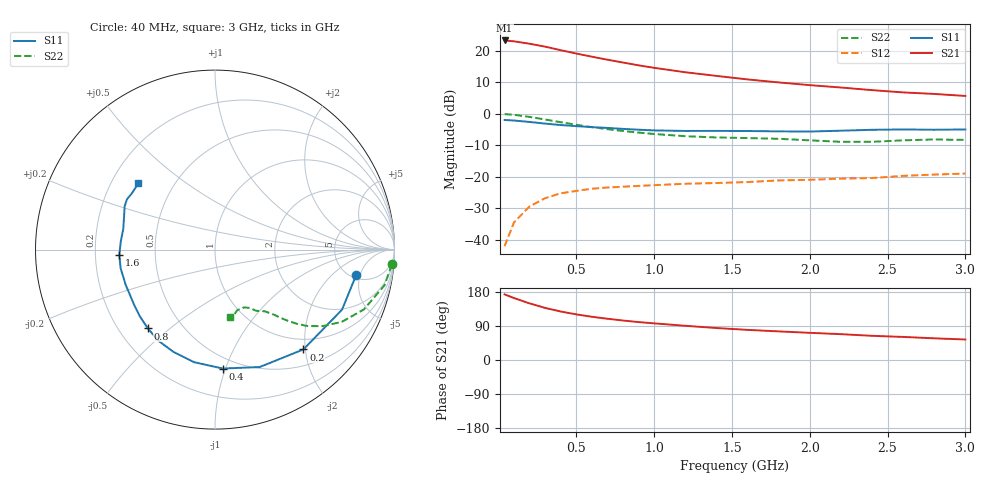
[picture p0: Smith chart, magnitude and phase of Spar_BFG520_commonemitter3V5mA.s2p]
! Filename:  BFG520B.S2P  Version:  2.1
! NXP part #: BFG520  Date: Feb 1992
! Bias condition: Vce=3V, Ic=5mA
! IN LINE PINNING: same data as with cross emitter pinning.
#  MHz  S  MA  R  50
! Freq  S11  S21  S12  S22  !GUM [dB]
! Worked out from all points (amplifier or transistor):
!   21 points, 40 MHz to 3 GHz, reference 50 ohm
!   highest |S21| = 23.2 dB at 40 MHz (marker M1)
!   |S21| within 3 dB of that: start of sweep to 393.2 MHz
!   unconditionally stable (mu >= 1): 1.746 GHz to end of sweep
!   at 300 MHz: K = 0.19, MSG = 24.0 dB, |S12| = -26.7 dB
!   at 1 GHz: K = 0.65, MSG = 18.6 dB, |S12| = -22.6 dB
!   at 3 GHz: K = 1.30, MAG = 9.0 dB, |S12| = -18.9 dB
!   lowest NFmin = 0.90 dB at 500 MHz
!   S11 on the Smith chart (normalised r, x): 40 MHz: 5.47, -4.32; 200 MHz: 0.79, -1.96; 400 MHz: 0.41, -0.98; 800 MHz: 0.32, -0.42; 1.6 GHz: 0.30, -0.03; 3 GHz: 0.31, +0.34
40  0.799 -10.3  14.52 173.1  0.008 84.1  0.989 -4.8
100  0.783 -25.3  14.07 163.5  0.019 77.0  0.965 -11.9
200  0.743 -48.5  12.89 149.4  0.034 66.6  0.894 -21.9
300  0.7 -69.2  11.59 137.5  0.046 58.1  0.813 -29.7
400  0.664 -86.3  10.19 128.0  0.055 52.3  0.736 -35.4
500  0.638 -100.5  9.02 120.4  0.06 47.6  0.67 -39.5
600  0.615 -112.1  8.033 114.1  0.065 44.7  0.615 -42.2
700  0.598 -121.7  7.204 108.9  0.068 42.6  0.571 -44.2
800  0.577 -130.4  6.491 104.2  0.07 41.7  0.535 -45.8
900  0.56 -138.4  5.868 100.1  0.072 41.1  0.504 -47.1
1000  0.546 -145.4  5.356 96.7  0.074 40.9  0.479 -48.4
1200  0.535 -158.4  4.556 90.3  0.078 40.6  0.442 -51.1
1400  0.536 -168.8  3.989 84.4  0.08 41.1  0.422 -54.0
1600  0.534 -176.7  3.507 79.5  0.083 43.4  0.413 -55.8
1800  0.527 175.3  3.144 75.5  0.088 44.4  0.402 -56.9
2000  0.524 167.1  2.847 71.7  0.09 46.6  0.38 -58.8
2200  0.54 159.7  2.61 68.2  0.094 47.7  0.36 -63.5
2400  0.558 154.5  2.372 63.8  0.096 50.1  0.36 -69.8
2600  0.565 150.3  2.183 60.9  0.104 51.9  0.38 -74.2
2800  0.559 145.5  2.065 57.2  0.109 52.4  0.392 -75.7
3000  0.565 139.3  1.918 54.1  0.113 54.8  0.386 -77.1
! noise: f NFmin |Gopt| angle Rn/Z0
500  0.9  0.396  29  0.24
900  1.1  0.334  50  0.26
1000  1.15  0.355  55  0.26
2000  1.85  0.275  130  0.16
